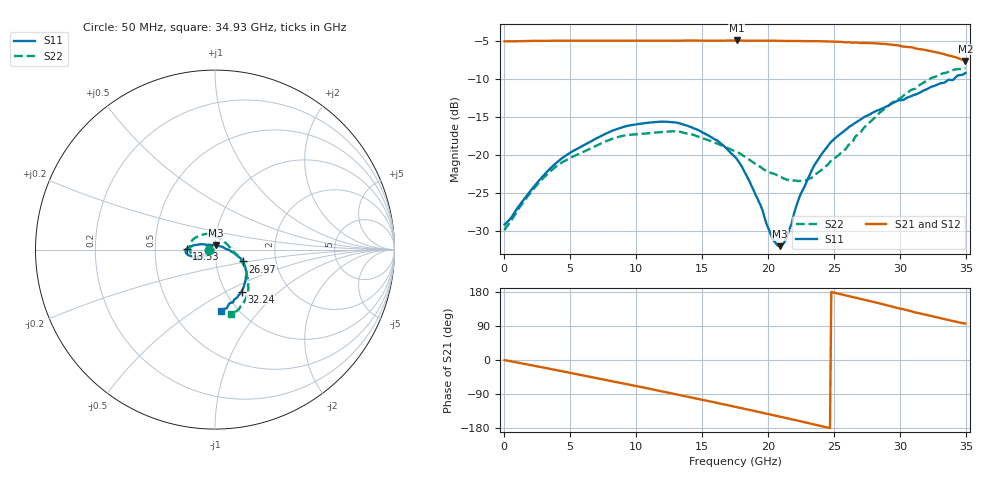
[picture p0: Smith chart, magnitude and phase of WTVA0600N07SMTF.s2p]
! 50 ohm 2-Port S-parameters measured by Modelithics Inc support@modelithics.com  Tampa, FL USA 813-866-6335 (February 2024)
! Smiths Interconnect,  6dB P/N: WTVA0600N07SMTF, Temperature: 50 C
! Board: 10 mil Rogers 4350B, Mounting Pad Dimensions: Length: 15 mils, Width: 25 mils, Gap: 40 mils.
# Hz S RI R 50
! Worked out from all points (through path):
!   352 points, 50 MHz to 34.93 GHz, reference 50 ohm
!   highest |S21| = -4.98 dB at 17.61 GHz (marker M1); lowest = -7.7 dB at 34.93 GHz (marker M2)
!   group delay of S21, straight-line fit = 21.1 ps
!   lowest |S11| = -32.1 dB at 20.9 GHz (marker M3), VSWR 1.05, Z = 50.4 + j2.48 ohm
!   |S11| at or under -10 dB: start of sweep to 34.1 GHz
!   |S22| runs from -30.0 to -8.6 dB; largest |S21 - S12| = 0.006
!   S11 on the Smith chart (normalised r, x): 50 MHz: 0.93, -0.00; 13.53 GHz: 0.73, +0.01; 26.97 GHz: 1.36, -0.18; 32.24 GHz: 1.18, -0.60; 34.93 GHz: 0.83, -0.65
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5e7  -0.0347 -0.000668  0.5557 -0.00276  0.5552 -0.00297  -0.0316 -0.00263
1.4935e9  -0.0466 -0.0194  0.5501 -0.0948  0.5496 -0.0947  -0.043 -0.0236
2.986e9  -0.0657 -0.0307  0.5269 -0.1911  0.5263 -0.1913  -0.0584 -0.039
4.18e9  -0.0836 -0.037  0.4946 -0.2651  0.494 -0.2649  -0.0722 -0.0476
5.8715e9  -0.1058 -0.04  0.4308 -0.36  0.4305 -0.3598  -0.0883 -0.0525
8.757e9  -0.1458 -0.0321  0.2808 -0.4853  0.28 -0.4851  -0.1253 -0.0394
1.1742e10  -0.1641 -0.0119  0.0879 -0.5536  0.0869 -0.5532  -0.1401 0.00555
1.3533e10  -0.1581 0.00495  -0.0384 -0.5611  -0.0394 -0.5605  -0.1322 0.0447
1.612e10  -0.1223 0.0223  -0.2202 -0.5171  -0.2205 -0.5163  -0.0905 0.0761
1.7513e10  -0.092 0.0278  -0.3107 -0.4695  -0.3105 -0.4689  -0.0613 0.0854
1.76125e10  -0.0893 0.0286  -0.3177 -0.4653  -0.317 -0.4649  -0.0588 0.0861
1.94035e10  -0.0384 0.0267  -0.4171 -0.3761  -0.4163 -0.3762  -0.012 0.0821
2.03985e10  -0.0107 0.0251  -0.4638 -0.3159  -0.4632 -0.3157  0.00654 0.0747
2.0896e10  0.00436 0.0246  -0.4831 -0.2829  -0.4825 -0.2826  0.0166 0.0695
2.1294e10  0.0175 0.0208  -0.4962 -0.2565  -0.4956 -0.2564  0.0236 0.0649
2.2289e10  0.0492 0.011  -0.5261 -0.1873  -0.526 -0.186  0.0437 0.0505
2.33835e10  0.0816 -0.00442  -0.5478 -0.1057  -0.5472 -0.1058  0.0638 0.0323
2.47765e10  0.1182 -0.028  -0.555 0.00503  -0.5544 0.00555  0.0914 0.00415
2.69655e10  0.156 -0.0657  -0.5146 0.1707  -0.5134 0.1722  0.1321 -0.043
2.91545e10  0.1736 -0.12  -0.4239 0.3198  -0.4207 0.3229  0.1744 -0.1205
3.2239e10  0.148 -0.2336  -0.2166 0.4296  -0.2144 0.43  0.1775 -0.2602
3.49255e10  0.031 -0.3426  -0.045 0.4108  -0.0452 0.4102  0.0916 -0.3604
